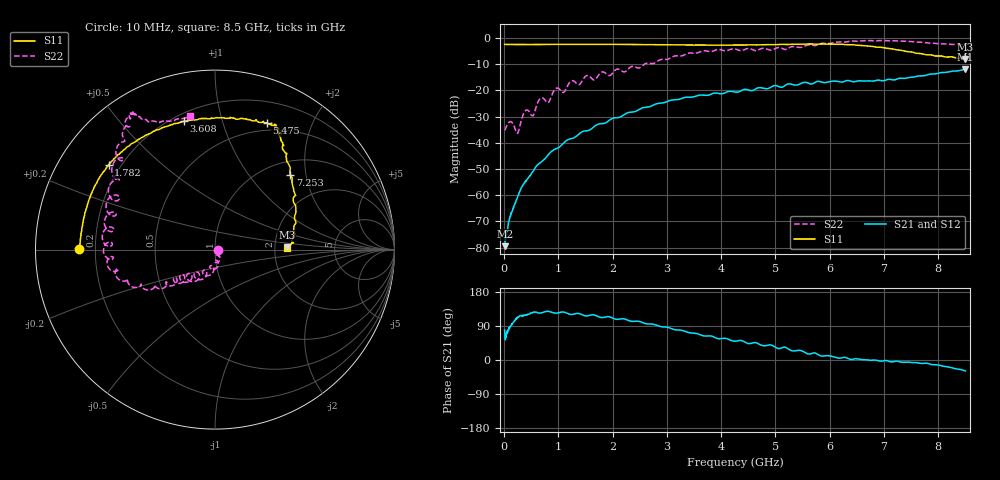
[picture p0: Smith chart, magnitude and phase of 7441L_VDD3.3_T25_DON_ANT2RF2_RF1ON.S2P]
!Agilent Technologies,E5071C,MY46417908,A.11.23
!Date: Mon May 03 19:53:38 2021
!Data & Calibration Information:
!Freq	S11:SOLT2(ON)	S21:SOLT2(ON)	S12:SOLT2(ON)	S22:SOLT2(ON)
!PortZ  Port1:50+j0  Port2:50+j0
!Above PortZ is port z conversion or system Z0 setting when saving the data.
!When reading, reference impedance value at option line is always used.
# Hz S dB R 50
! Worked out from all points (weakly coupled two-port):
!   1601 points, 10 MHz to 8.5 GHz, reference 50 ohm
!   highest |S21| = -12.01 dB at 8.5 GHz (marker M1); lowest = -79.5 dB at 15.31 MHz (marker M2)
!   lowest |S11| = -8.0 dB at 8.489 GHz (marker M3), VSWR 2.33, Z = 116 + j3.41 ohm
!   |S11| at or under -10 dB: nowhere
!   |S22| runs from -36.4 to -0.9 dB; largest |S21 - S12| = 0.0056
!   S11 on the Smith chart (normalised r, x): 10 MHz: 0.14, +0.00; 1.782 GHz: 0.15, +0.34; 3.608 GHz: 0.24, +0.76; 5.475 GHz: 0.42, +1.40; 7.253 GHz: 1.28, +1.63; 8.5 GHz: 2.33, +0.05
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1e7  -2.41 179.6  -79.08 79.1  -79.74 50.9  -35.16 -0.6
1.530625e7  -2.43 179.5  -79.45 66.9  -79.78 54.8  -35.07 -0.7
1.214312e8  -2.47 176.8  -67.89 89.6  -67.65 89.1  -31.90 -36.2
2.487812e8  -2.49 173.6  -60.79 111.5  -60.70 112.0  -36.38 -44.8
3.9205e8  -2.49 169.9  -54.85 118.5  -54.85 117.9  -27.75 -58.6
5.247062e8  -2.47 166.8  -51.08 124.8  -51.03 125.3  -29.71 -70.3
6.67975e8  -2.47 163.6  -47.57 124.3  -47.58 124.2  -23.02 -74.4
8.643062e8  -2.45 159.1  -43.43 126.8  -43.42 126.6  -22.64 -76.2
9.598188e8  -2.43 157.1  -42.28 123.6  -42.22 123.3  -19.17 -92.5
1.092475e9  -2.43 154.5  -40.20 126.6  -40.17 126.4  -20.76 -101.4
1.235744e9  -2.41 151.8  -38.44 120.1  -38.39 120.2  -16.42 -105.7
1.426769e9  -2.40 148.3  -35.91 120.4  -35.88 120.4  -16.79 -108.6
1.782288e9  -2.42 141.5  -32.74 112.2  -32.70 112.3  -13.19 -125.2
2.843538e9  -2.57 120.3  -24.94 89.8  -24.96 89.9  -8.62 -144.0
3.607638e9  -2.67 103.6  -21.78 67.0  -21.80 67.0  -5.29 -161.2
4.255e9  -2.67 89.1  -20.62 49.6  -20.64 49.3  -4.19 178.4
5.475438e9  -2.36 67.9  -17.28 24.7  -17.27 25.1  -3.55 144.3
5.671769e9  -2.28 66.0  -17.53 17.5  -17.53 17.4  -2.70 135.7
7.088538e9  -4.00 49.9  -15.73 -3.4  -15.70 -3.2  -1.05 121.3
7.253031e9  -4.57 44.7  -15.56 -3.2  -15.54 -3.0  -1.14 120.6
8.489388e9  -7.97 1.8  -12.03 -28.4  -11.87 -27.8  -2.47 101.2
8.5e9  -7.96 1.3  -12.01 -28.9  -11.85 -28.4  -2.44 100.7
